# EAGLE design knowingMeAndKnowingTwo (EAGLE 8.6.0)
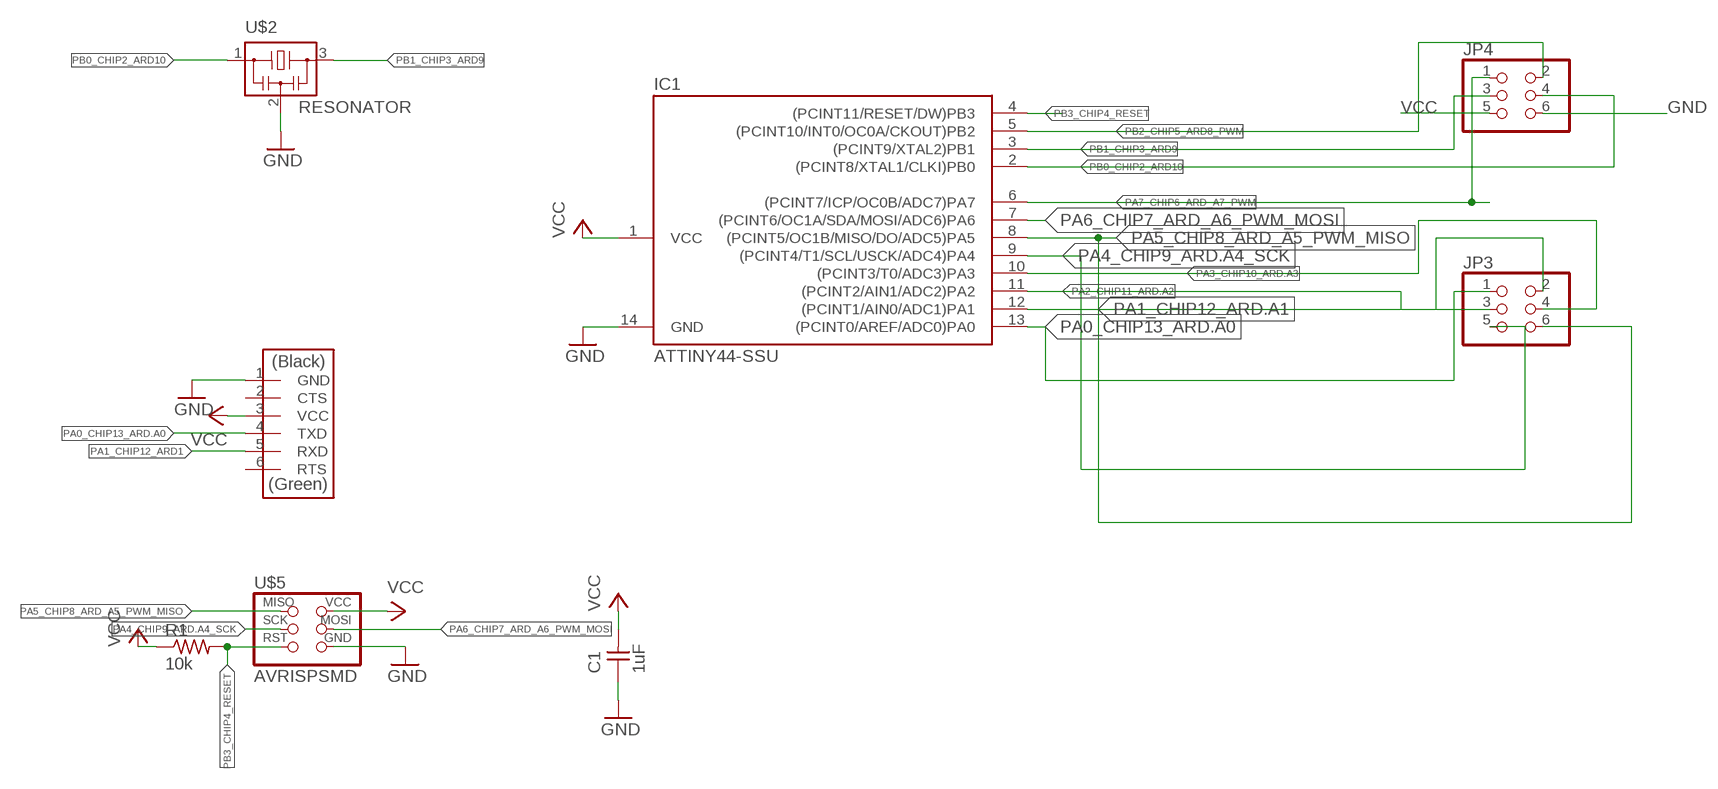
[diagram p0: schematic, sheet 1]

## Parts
C1  1uF  CAP-UNPOLARIZEDFAB  [C1206FAB]
IC1  ATTINY44-SSU  [SOIC14]
JP3  PINHD-2X03_2.54-SMD  [2X03SMD]
JP4  PINHD-2X03_2.54-SMD  [2X03SMD]
R1  10k  RES-US1206FAB  [R1206FAB]
U$2  RESONATOR  [EFOBM]
U$3  FTDI-SMD-HEADER  [1X06SMD]
U$5  AVRISPSMD  [2X03SMD]

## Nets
GND: C1.1 IC1.14(GND) JP4.6 U$2.2 U$3.1(GND) U$5.6(GND)
PA0_CHIP13_ARD.A0: IC1.13((PCINT0/AREF/ADC0)PA0) JP3.1 U$3.4(TXD)
PA1_CHIP12_ARD1: U$3.5(RXD)
PA1_CHIP12_ARD.A1: IC1.12((PCINT1/AIN0/ADC1)PA1) JP3.2
PA2_CHIP11_ARD.A2: IC1.11((PCINT2/AIN1/ADC2)PA2) JP3.3
PA3_CHIP10_ARD.A3: IC1.10((PCINT3/T0/ADC3)PA3) JP3.4
PA4_CHIP9_ARD.A4_SCK: IC1.9((PCINT4/T1/SCL/USCK/ADC4)PA4) JP3.5 U$5.3(SCK)
PA5_CHIP8_ARD_A5_PWM_MISO: IC1.8((PCINT5/OC1B/MISO/DO/ADC5)PA5) JP3.6 U$5.1(MISO)
PA6_CHIP7_ARD_A6_PWM_MOSI: IC1.7((PCINT6/OC1A/SDA/MOSI/ADC6)PA6) U$5.4(MOSI)
PA7_CHIP6_ARD_A7_PWM: IC1.6((PCINT7/ICP/OC0B/ADC7)PA7) JP4.1
PB0_CHIP2_ARD10: IC1.2((PCINT8/XTAL1/CLKI)PB0) JP4.4 U$2.1
PB1_CHIP3_ARD9: IC1.3((PCINT9/XTAL2)PB1) JP4.3 U$2.3
PB2_CHIP5_ARD8_PWM: IC1.5((PCINT10/INT0/OC0A/CKOUT)PB2) JP4.2
PB3_CHIP4_RESET: IC1.4((PCINT11/RESET/DW)PB3) R1.2 U$5.5(RST)
VCC: C1.2 IC1.1(VCC) JP4.5 R1.1 U$3.3(VCC) U$5.2(VCC)
Unconnected: U$3.2(CTS) U$3.6(RTS)

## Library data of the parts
C1 = fab:CAP-UNPOLARIZED
IC1 = fab:ATTINY44
JP3 JP4 = pinhead-2:PINHD-2X03: PIN HEADER
R1 = fab:RES-US: Resistor (US Symbol)
U$2 = fab:RESONATOR
U$3 = fab:FTDI-SMD-HEADER
U$5 = fab:AVRISP

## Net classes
0 default: width 0.3 mm, clearance 0.4 mm

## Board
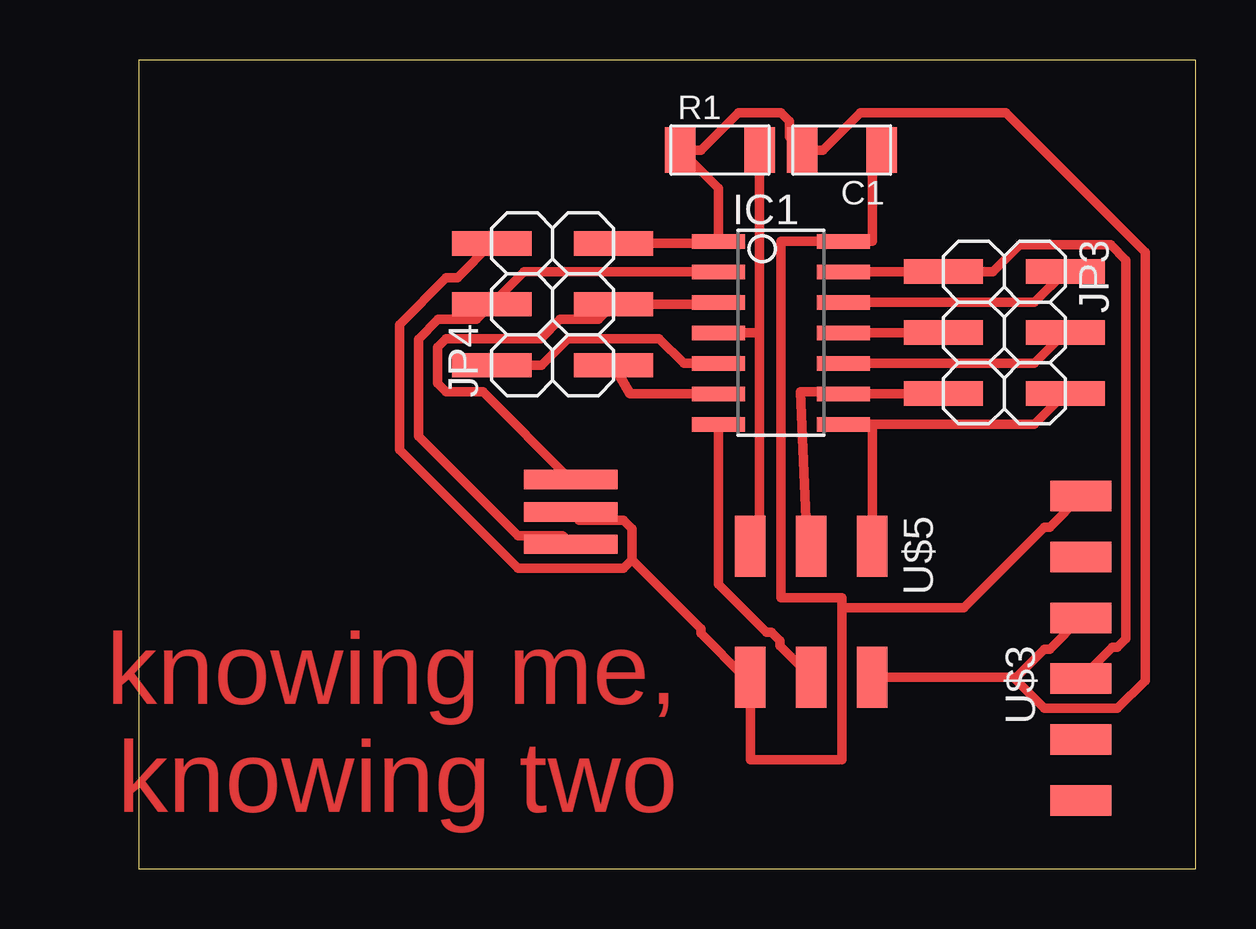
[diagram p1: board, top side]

Size 44.07 x 33.69 mm. Coordinates in mm from the lower left corner, seen from the top.
Outline: 0,0 44.07,0 44.07,33.69 0,33.69 0,0
Copper layers (1*16): Top 0.035mm / dielectric 1.5mm / Bottom 0.035mm
Design rules "default *": minimum track width 0.3mm, minimum drill 0.8mm, track to track 0.4mm, track to pad 0.4mm, pad to pad 0.4mm, via to via 0.4mm, smd to smd 6mil, copper to edge 40mil, drill to drill 6mil, minimum pad ring 10mil, minimum via ring 8mil, stop-mask expansion 4mil, vias tented up to drill 0mil, thermal gap 10mil

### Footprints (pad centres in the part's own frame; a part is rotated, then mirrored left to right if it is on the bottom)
C1206FAB = smd 1.27 x 1.905: 1 -1.651,0; 2 1.651,0
SOIC14 = smd 0.61 x 2.21: 1 -3.81,-2.603; 2 -2.54,-2.603; 3 -1.27,-2.603; 4 0,-2.603; 5 1.27,-2.603; 6 2.54,-2.603; 7 3.81,-2.603; 8 3.81,2.603; 9 2.54,2.603; 10 1.27,2.603; 11 0,2.603; 12 -1.27,2.603; 13 -2.54,2.603; 14 -3.81,2.603
2X03SMD = smd 1.016 x 3.302: 1 -1.27,-3.81; 2 -1.27,1.27; 3 1.27,-3.81; 4 1.27,1.27; 5 3.81,-3.81; 6 3.81,1.27
R1206FAB = smd 1.27 x 1.905: 1 -1.651,0; 2 1.651,0
EFOBM = smd 0.8 x 3.9: 1 -1.35,0; 2 0,0; 3 1.35,0
1X06SMD = smd 2.54 x 1.27: 1 0,6.35; 2 0,3.81; 3 0,1.27; 4 0,-1.27; 5 0,-3.81; 6 0,-6.35
2X03SMD' = smd 2.54 x 1.27: 1 -2.54,2.54; 2 2.92,2.54; 3 -2.54,0; 4 2.92,0; 5 -2.54,-2.54; 6 2.92,-2.54

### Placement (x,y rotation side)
C1  29.31,29.94 180 top
IC1  26.77,22.32 270 top
JP3  37.35,23.61 270 top
JP4  15.99,22.24 90 top
R1  24.23,29.94 0 top
U$2  18.01,14.86 90 top
U$3  39.28,9.18 0 top
U$5  AVRISPSMD  [2X03SMD']  28.04,10.89 270 top

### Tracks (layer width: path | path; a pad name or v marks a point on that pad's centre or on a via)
GND
  Top 0.4: C1.1 30.58,29.56 30.58,26.13 IC1.14 26.77,26.13 26.77,11.29 29.31,11.29 29.31,10.86 | 29.31,4.54 29.31,4.66 | 29.31,4.66 29.31,10.86 | 29.31,4.66 29.19,4.54 25.5,4.54 U$5.6 25.26,7.97 23.43,9.8 23.43,9.99 20.56,12.86 | 20.56,12.86 20.56,14.16 20.21,14.51 18.36,14.51 U$2.2 | 20.56,12.86 20.21,12.51 15.81,12.51 10.87,17.45 10.87,22.67 12.82,24.62 13.29,24.62 JP4.6 | U$3.1 37.98,14.22 37.76,14.22 34.4,10.86 29.31,10.86
PA0_CHIP13_ARD.A0
  Top 0.4: IC1.13 29.39,24.88 JP3.1 35.61,24.88 36.72,25.98 40.52,25.98 41.15,25.36 41.15,9.57 40.8,9.21 40.59,9.21 U$3.4
PA1_CHIP12_ARD.A1
  Top 0.4: IC1.12 37.34,23.59 JP3.2
PA2_CHIP11_ARD.A2
  Top 0.4: IC1.11 33.53,22.32 JP3.3
PA3_CHIP10_ARD.A3
  Top 0.4: IC1.10 37.34,21.05 JP3.4
PA4_CHIP9_ARD.A4_SCK
  Top 0.4: U$5.3 27.86,13.61 27.59,19.86 29.29,19.86 IC1.9 33.53,19.78 JP3.5
PA5_CHIP8_ARD_A5_PWM_MISO
  Top 0.4: 30.94,13.79 U$5.1 30.58,18.51 IC1.8 37.34,18.51 JP3.6
PA6_CHIP7_ARD_A6_PWM_MOSI
  Top 0.4: U$5.4 26.73,9.27 26.73,9.49 26.38,9.84 26.17,9.84 24.17,11.84 IC1.7
PA7_CHIP6_ARD_A7_PWM
  Top 0.4: JP4.1 20.48,19.78 IC1.6
PB0_CHIP2_ARD10
  Top 0.4: IC1.2 16.07,24.86 JP4.4 14.08,22.88 12.49,22.88 11.67,22.06 11.67,18 15.81,13.86 17.66,13.86 U$2.1
PB1_CHIP3_ARD9
  Top 0.4: IC1.3 24.09,23.51 JP4.3 19.16,22.88 17.57,22.88 16.77,22.08 12.82,22.08 12.47,21.73 12.47,20.21 12.82,19.86 14.36,19.86 U$2.3
PB2_CHIP5_ARD8_PWM
  Top 0.4: JP4.2 16.79,20.97 17.9,22.08 21.7,22.08 22.73,21.05 IC1.5
PB3_CHIP4_RESET
  Top 0.4: R1.2 25.88,22.32 | 25.88,22.32 25.88,14.26 | 25.88,14.26 25.88,13.81 | IC1.4 25.88,22.32 | U$5.5 25.5,13.88 25.88,14.26
VCC
  Top 0.4: JP4.5 24.09,26.05 IC1.1 24.17,28.35 R1.1 23.45,29.94 25,31.49 26.77,31.49 27.12,31.14 27.12,30.48 C1.2 28.52,29.94 30.08,31.49 36.14,31.49 41.95,25.69 41.95,7.83 40.8,6.68 37.76,6.68 36.47,7.97 U$5.2 36.59,7.97 37.76,9.14 37.98,9.14 U$3.3

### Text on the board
Top: knowing me, / knowing two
